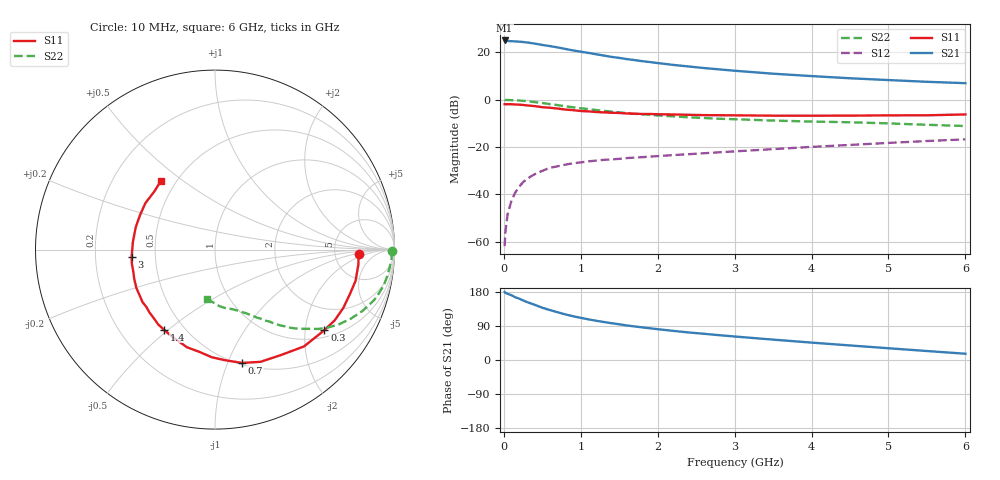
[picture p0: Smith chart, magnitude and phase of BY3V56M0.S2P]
! SIEMENS Small Signal Semiconductors
! BFY420
! Si NPN RF SIEGET Grounded Emitter Transistor in MICRO-X
! VCE = 3.5 V  IC = 6 mA
! Common Emitter S-Parameters:  October  1996
# GHz  S  MA  R  50
!  f  S11  S21  S12  S22
! GHz  MAG  ANG  MAG  ANG  MAG  ANG  MAG  ANG
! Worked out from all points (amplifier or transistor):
!   36 points, 10 MHz to 6 GHz, reference 50 ohm
!   highest |S21| = 25.0 dB at 10 MHz (marker M1)
!   |S21| within 3 dB of that: start of sweep to 708.8 MHz
!   unconditionally stable (mu >= 1): 3 GHz to end of sweep
!   at 250 MHz: K = 0.15, MSG = 29.6 dB, |S12| = -34.9 dB
!   at 1.4 GHz: K = 0.58, MSG = 21.7 dB, |S12| = -25.3 dB
!   at 6 GHz: K = 1.12, MAG = 9.8 dB, |S12| = -16.8 dB
!   S11 on the Smith chart (normalised r, x): 10 MHz: 9.06, -1.15; 300 MHz: 1.20, -2.53; 700 MHz: 0.52, -1.13; 1.4 GHz: 0.39, -0.48; 3 GHz: 0.36, -0.04; 6 GHz: 0.41, +0.42
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0.01  0.8041 -1.6  17.88 179.6  0.0008 51.3  0.9853 -0.6
0.02  0.8006 -2.7  17.8 177.3  0.0016 65.1  0.9835 -1.1
0.05  0.8032 -6.0  17.37 174.6  0.0039 80.7  0.9855 -3.0
0.1  0.8023 -12.5  17.25 170.9  0.0074 80.1  0.9775 -6.1
0.15  0.7912 -18.4  17.05 165.4  0.011 77.1  0.9697 -9.2
0.2  0.7854 -24.5  16.86 161.9  0.0145 77.1  0.9608 -12.0
0.3  0.757 -36.4  16.22 153.0  0.0213 70.6  0.9303 -17.6
0.4  0.7328 -47.4  15.36 145.8  0.0265 65.9  0.89 -22.6
0.5  0.6937 -57.7  14.36 137.9  0.0313 62.5  0.8486 -27.0
0.6  0.6748 -67.9  13.58 131.7  0.0363 58.1  0.8072 -31.0
0.7  0.6494 -76.5  12.74 125.9  0.0391 55.4  0.767 -34.4
0.8  0.6192 -84.7  11.83 120.3  0.0424 51.9  0.7263 -37.5
0.9  0.6004 -91.6  11.02 115.5  0.0452 49.9  0.6909 -39.7
1.1  0.5662 -106.0  9.744 107.3  0.0496 47.2  0.6305 -44.2
1.4  0.5287 -122.6  8.032 97.1  0.0546 44.4  0.5598 -49.1
1.7  0.5059 -136.2  6.864 88.6  0.0597 42.6  0.5022 -52.9
2.2  0.4875 -153.9  5.442 76.9  0.0673 41.2  0.4445 -58.4
3  0.4669 -174.7  4.092 62.0  0.0808 39.8  0.3863 -65.4
3.5  0.4593 174.4  3.545 53.8  0.09 38.6  0.362 -69.7
4.5  0.46 154.9  2.837 38.4  0.1106 34.5  0.3333 -79.2
5.5  0.4678 136.5  2.388 23.7  0.1337 28.8  0.2946 -91.9
6  0.4874 128.0  2.235 16.5  0.1451 25.2  0.2776 -99.8
